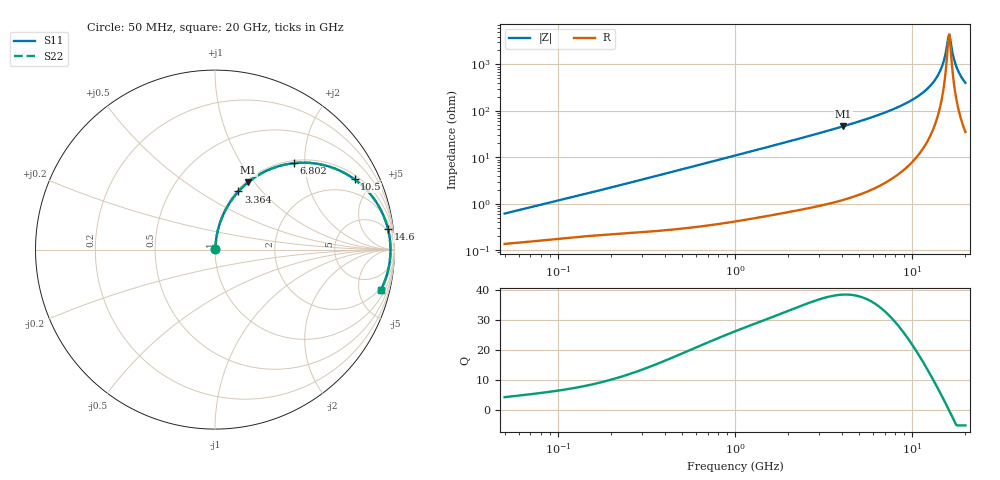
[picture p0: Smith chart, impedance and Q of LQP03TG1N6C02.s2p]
!Murata Part Number: LQP03TG1N6C02
!These Parameters are Measured in Series Mode Connection
!  o--[Z]--o
!Port1  Port2
!  o-------o
!Freq. Start=50[MHz] Stop=20[GHz], 401[Steps]
# Hz S RI R 50
!Freq.(Hz) S11(Real) S11(Imag) S21(Real) S21(Imag) S12(Real) S12(Imag) S22(Real) S22(Imag)
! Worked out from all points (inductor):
!   401 points, 50 MHz to 20 GHz, reference 50 ohm
!   read as one part in series: L = 1.89 nH near 51.52 MHz
!   highest Q = 38.4 at 4.088 GHz (marker M1), where L = 1.82 nH
!   self-resonance near 15.98 GHz
!   S11 on the Smith chart (normalised r, x): 50 MHz: 1.00, +0.01; 3.364 GHz: 1.02, +0.75; 6.802 GHz: 1.05, +1.76; 10.5 GHz: 1.19, +3.86; 14.6 GHz: 4, +16; 20 GHz: 1.70, -8.04
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5e7  0.00141 0.006  0.9986 -0.006  0.9986 -0.006  0.00141 0.006
1.364002e8  0.00221 0.0155  0.9978 -0.0155  0.9978 -0.0155  0.00221 0.0155
3.721004e8  0.0043 0.0409  0.9957 -0.0409  0.9957 -0.0409  0.0043 0.0409
1e9  0.0158 0.1071  0.9842 -0.1071  0.9842 -0.1071  0.0158 0.1071
2.728004e9  0.0896 0.2721  0.9104 -0.2721  0.9104 -0.2721  0.0896 0.2721
3.364474e9  0.1308 0.3241  0.8692 -0.3241  0.8692 -0.3241  0.1308 0.3241
4.087748e9  0.1854 0.3758  0.8146 -0.3758  0.8146 -0.3758  0.1854 0.3758
6.802353e9  0.439 0.4816  0.561 -0.4816  0.561 -0.4816  0.439 0.4816
7.442007e9  0.5031 0.4843  0.4969 -0.4843  0.4969 -0.4843  0.5031 0.4843
1.050288e10  0.7773 0.3917  0.2227 -0.3917  0.2227 -0.3917  0.7773 0.3917
1.276073e10  0.9093 0.2472  0.0907 -0.2472  0.0907 -0.2472  0.9093 0.2472
1.375312e10  0.9446 0.1751  0.0554 -0.1751  0.0554 -0.1751  0.9446 0.1751
1.460232e10  0.9642 0.1128  0.0358 -0.1128  0.0358 -0.1128  0.9642 0.1128
1.504638e10  0.9709 0.0805  0.0291 -0.0805  0.0291 -0.0805  0.9709 0.0805
1.573793e10  0.9768 0.0312  0.0232 -0.0312  0.0232 -0.0312  0.9768 0.0312
1.597544e10  0.9777 0.0147  0.0223 -0.0147  0.0223 -0.0147  0.9777 0.0147
1.621653e10  0.978 -0.00194  0.022 0.00194  0.022 0.00194  0.978 -0.00194
1.646126e10  0.9777 -0.0185  0.0223 0.0185  0.0223 0.0185  0.9777 -0.0185
1.721783e10  0.9735 -0.0681  0.0265 0.0681  0.0265 0.0681  0.9735 -0.0681
1.800918e10  0.9643 -0.1168  0.0357 0.1168  0.0357 0.1168  0.9643 -0.1168
1.912117e10  0.9446 -0.1793  0.0554 0.1793  0.0554 0.1793  0.9446 -0.1793
2e10  0.9248 -0.2235  0.0752 0.2235  0.0752 0.2235  0.9248 -0.2235
